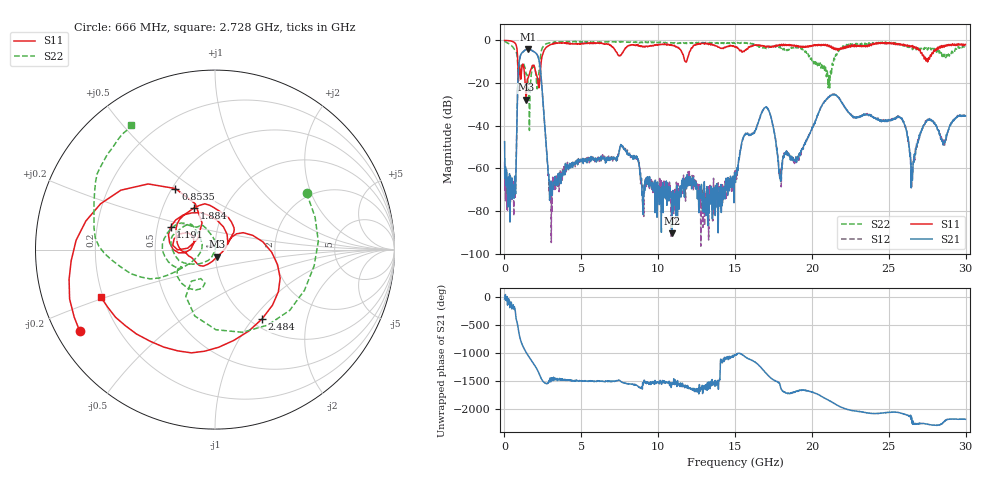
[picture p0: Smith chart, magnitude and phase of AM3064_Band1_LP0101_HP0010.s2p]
# Hz S DB R 50.0
!freq dBS11 angS11 dBS21 angS21 dBS12 angS12 dBS22 angS22
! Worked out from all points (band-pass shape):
!   1600 points, 10 MHz to 29.98 GHz, reference 50 ohm
!   highest |S21| = -4.16 dB at 1.528 GHz (marker M1); lowest = -90.5 dB at 10.88 GHz (marker M2)
!   |S21| within 3 dB of the highest: 1.04 GHz to 2.156 GHz (1.116 GHz wide, 69.8 % of centre)
!   lowest |S11| = -27.8 dB at 1.416 GHz (marker M3), VSWR 1.09, Z = 51.1 - j4 ohm
!   |S11| at or under -10 dB: 865.9 MHz to 2.391 GHz (1.525 GHz wide, 93.6 % of centre); 11.77 GHz to 11.84 GHz (67.24 MHz wide, 0.569 % of centre); 27.52352 GHz to 27.53402 GHz (10.5 MHz wide, 0.0382 % of centre)
!   |S22| runs from -42.2 to -0.4 dB; largest |S21 - S12| = 0.0071
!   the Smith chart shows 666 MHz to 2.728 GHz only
!   S11 on the Smith chart (normalised r, x): 666 MHz: 0.07, -0.28; 853.5 MHz: 0.52, +0.42; 1.191 GHz: 0.59, +0.16; 1.884 GHz: 0.72, +0.36; 2.484 GHz: 1.13, -1.11; 2.728 GHz: 0.19, -0.19
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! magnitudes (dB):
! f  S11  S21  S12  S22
! 10 MHz  0.0  -47.5  -56.9  -0.4
! 666 MHz  -1.1  -63.6  -67.1  -4.4
! 853.5 MHz  -7.8  -24.6  -24.5  -10.3
! 1.191 GHz  -11.1  -5.5  -5.5  -10.7
! 1.416 GHz  -27.8  -4.3  -4.3  -15.9
! 1.528 GHz  -17.8  -4.2  -4.1  -19.1
! 1.884 GHz  -11.7  -5.1  -5.2  -12.0
! 2.484 GHz  -6.6  -26.3  -26.3  -3.3
! 2.728 GHz  -3.2  -50.5  -50.0  -1.6
! 3.046 GHz  -1.9  -66.3  -94.8  -1.0
! 5.015 GHz  -1.5  -56.7  -55.5  -0.7
! 10 GHz  -2.0  -73.5  -73.4  -0.9
! 10.88 GHz  -2.4  -90.5  -75.0  -1.2
! 15 GHz  -3.1  -63.3  -61.1  -1.4
! 16.94 GHz  -2.7  -31.6  -31.5  -3.6
! 17.93 GHz  -2.0  -64.9  -64.8  -2.9
! 19.99 GHz  -2.8  -41.7  -42.0  -9.4
! 21.38 GHz  -3.2  -25.6  -25.4  -11.6
! 25 GHz  -1.1  -37.6  -37.2  -1.1
! 26.53 GHz  -2.5  -65.6  -60.7  -4.3
! 27.51 GHz  -9.3  -37.3  -37.3  -4.4
! 29.98 GHz  -1.9  -35.4  -35.7  -2.9
